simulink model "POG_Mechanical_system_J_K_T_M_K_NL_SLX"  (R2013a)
settings: Solver=ode45  StartTime=0.0  StopTime=10.0  MaxStep=0.001  RelTol=1e-3
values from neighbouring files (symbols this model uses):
  b_1 = 1*Nm/(10*rpm)    (= 0.954929658551)    [POG_Mechanical_system_J_K_T_M_K_Par_SLX_m.m]    (also in POG_Mechanical_system_J_K_T_M_K_SLX_m.m = 1; POG_Mechanical_system_J_K_T_M_K_SuperBlock_SLX_m.m = 1; POG_Mechanical_system_J_K_T_M_K_NL_SLX_m.m)
  F_out = [-K_1*x_b -x_b x_b K_1*x_b]    [POG_Mechanical_system_J_K_T_M_K_NL_SLX_m.m]
  J = 1*kg*(30*cm)^2    (= 0.09)    [POG_Mechanical_system_J_K_T_M_K_Par_SLX_m.m]    (also in POG_Mechanical_system_J_K_T_M_K_SLX_m.m = 1; POG_Mechanical_system_J_K_T_M_K_SuperBlock_SLX_m.m = 1; POG_Mechanical_system_J_K_T_M_K_NL_SLX_m.m)
  K_2 = 20*Newton/(1*cm)    (= 2000)    [POG_Mechanical_system_J_K_T_M_K_Par_SLX_m.m]    (also in POG_Mechanical_system_J_K_T_M_K_SLX_m.m = 1; POG_Mechanical_system_J_K_T_M_K_SuperBlock_SLX_m.m = 1; POG_Mechanical_system_J_K_T_M_K_NL_SLX_m.m)
  Nc = 30*Newton    (= 30)    [POG_Mass_Linear_Control_SLX_m.m]    (also in POG_Mechanical_system_J_K_T_M_K_NL_SLX_m.m = 2)
  P_2_0 = 0    [POG_Mechanical_system_J_K_T_M_K_Par_SLX_m.m]    (also in POG_Mechanical_system_J_K_T_M_K_SLX_m.m; POG_Mechanical_system_J_K_T_M_K_SuperBlock_SLX_m.m; POG_Mechanical_system_J_K_T_M_K_NL_SLX_m.m)
  Ph_T = pi/2    (= 1.57079632679)    [POG_Mechanical_system_J_K_T_M_K_NL_SLX_m.m]
  R = 40*cm    (= 0.4)    [POG_Mechanical_system_J_K_T_M_K_Par_SLX_m.m]    (also in POG_Mechanical_system_J_K_T_M_K_SLX_m.m = 1; POG_Mechanical_system_J_K_T_M_K_SuperBlock_SLX_m.m = 1; POG_Mechanical_system_J_K_T_M_K_NL_SLX_m.m)
  T = 10*Nm    (= 10)    [POG_Mechanical_system_J_K_T_M_K_Par_SLX_m.m]    (also in POG_Mechanical_system_J_K_T_M_K_SLX_m.m; POG_Mechanical_system_J_K_T_M_K_SuperBlock_SLX_m.m; POG_Mechanical_system_J_K_T_M_K_NL_SLX_m.m = 2)
  Ts = Tfin/Nr_Ts_Points    (= 0.0025)    [POG_Mechanical_system_J_K_T_M_K_Par_SLX_m.m]    (also in POG_Mechanical_system_J_K_T_M_K_SLX_m.m = 0.005; POG_Mechanical_system_J_K_T_M_K_SuperBlock_SLX_m.m = 0.005; POG_Mass_Linear_Control_SLX_m.m; POG_Mechanical_system_J_K_T_M_K_NL_SLX_m.m)
  v_d = 0    [POG_Mechanical_system_J_K_T_M_K_Par_SLX_m.m]    (also in POG_Mechanical_system_J_K_T_M_K_SLX_m.m; POG_Mechanical_system_J_K_T_M_K_SuperBlock_SLX_m.m; POG_Mechanical_system_J_K_T_M_K_NL_SLX_m.m)
  Vx0 = 0    [POG_Mechanical_system_J_K_T_M_K_NL_SLX_m.m]
  w_T = 2*pi*1    (= 6.28318530718)    [POG_Mechanical_system_J_K_T_M_K_NL_SLX_m.m]
  x_6_0 = 0    [POG_Mechanical_system_J_K_T_M_K_Par_SLX_m.m]    (also in POG_Mechanical_system_J_K_T_M_K_SLX_m.m; POG_Mechanical_system_J_K_T_M_K_SuperBlock_SLX_m.m; POG_Mechanical_system_J_K_T_M_K_NL_SLX_m.m)
  x_9_0 = 0    [POG_Mechanical_system_J_K_T_M_K_Par_SLX_m.m]    (also in POG_Mechanical_system_J_K_T_M_K_SLX_m.m; POG_Mechanical_system_J_K_T_M_K_SuperBlock_SLX_m.m; POG_Mechanical_system_J_K_T_M_K_NL_SLX_m.m)
  X_in = [  -2*x_b -x_b x_b   2*x_b]    [POG_Mechanical_system_J_K_T_M_K_NL_SLX_m.m]
undefined symbols (not defined in the file or in its folder): b, m

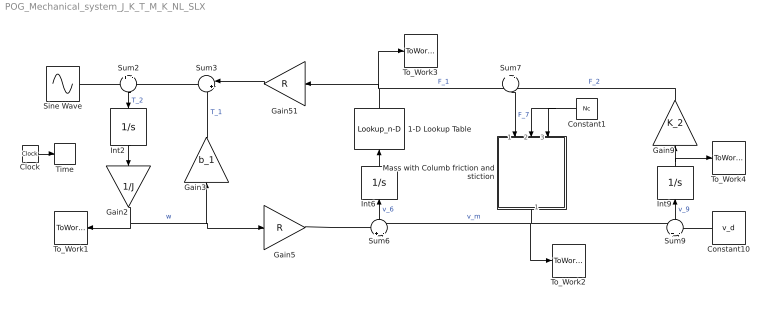
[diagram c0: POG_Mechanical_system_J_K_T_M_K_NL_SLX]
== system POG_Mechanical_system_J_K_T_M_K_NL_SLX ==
  1-D Lookup Table : Lookup_n-D  NumberOfTableDimensions=1  BreakpointsForDimension1=X_in  Table=F_out  RndMeth=Simplest
  Clock : Clock
  Constant1 : Constant  Value=Nc
  Constant10 : Constant  Value=v_d
  Gain2 : Gain  Gain=1/J
  Gain3 : Gain  Gain=b_1
  Gain5 : Gain  Gain=R
  Gain51 : Gain  Gain=R
  Gain9 : Gain  Gain=K_2
  Int2 : Integrator  InitialCondition=P_2_0
  Int6 : Integrator  InitialCondition=x_6_0
  Int9 : Integrator  InitialCondition=x_9_0
  Mass with Columb friction and stiction : Subsystem
  Sine Wave : Sin  Amplitude=T  Frequency=w_T  Phase=Ph_T  SampleTime=0
  Sum{2,6..7,9} (4 alike) : Sum  Inputs=+|-
  Sum3 : Sum  Inputs=|++
  Time : ToWorkspace  VariableName=t  SampleTime=Ts
  To_Work1 : ToWorkspace  VariableName=w_1  SampleTime=Ts
  To_Work2 : ToWorkspace  VariableName=w_m  SampleTime=Ts
  To_Work3 : ToWorkspace  VariableName=F_1  SampleTime=Ts
  To_Work4 : ToWorkspace  VariableName=x  SampleTime=Ts
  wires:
  Sine Wave/1 -> Sum2/1
  Sum3/1 -> Sum2/2
  Gain2/1 -> To_Work1/1, Gain3/1, Gain5/1  "w"
  Sum2/1 -> Int2/1  "T_2"
  Int2/1 -> Gain2/1
  Gain51/1 -> Sum3/1
  Gain3/1 -> Sum3/2  "T_1"
  Gain5/1 -> Sum6/1
  1-D Lookup Table/1 -> To_Work3/1, Gain51/1, Sum7/1  "F_1"
  Mass with Columb friction and stiction/1(Vx) -> Sum6/2, To_Work2/1, Sum9/1  "v_m"
  Sum6/1 -> Int6/1  "v_6"
  Int6/1 -> 1-D Lookup Table/1
  Sum7/1 -> Mass with Columb friction and stiction/1(F)  "F_7"
  Gain9/1 -> Sum7/2  "F_2"
  Constant10/1 -> Sum9/2
  Sum9/1 -> Int9/1  "v_9"
  Int9/1 -> To_Work4/1, Gain9/1
  Clock/1 -> Time/1
  Constant1/1 -> Mass with Columb friction and stiction/3(Ns), Mass with Columb friction and stiction/2(Nc)

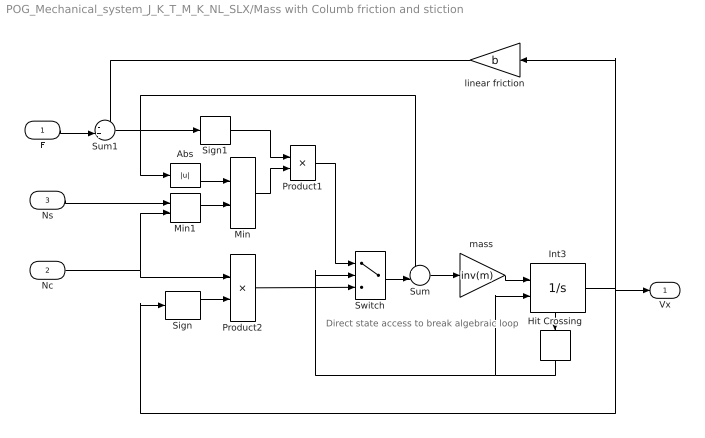
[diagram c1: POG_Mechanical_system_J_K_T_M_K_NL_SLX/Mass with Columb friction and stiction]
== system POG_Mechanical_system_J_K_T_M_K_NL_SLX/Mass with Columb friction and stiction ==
  note: Direct state access to break algebraic loop
  F : Inport
  Nc : Inport  Port=2
  Ns : Inport  Port=3
  Abs : Abs
  Hit Crossing : HitCross
  Int3 : Integrator  ExternalReset=rising  InitialCondition=Vx0  ShowStatePort=on
  Min : MinMax  Inputs=2
  Min1 : MinMax  Function=max  Inputs=2
  Product1 : Product
  Product2 : Product
  Sign : Signum
  Sign1 : Signum
  Sum : Sum  Inputs=+-|
  Sum1 : Sum  Inputs=-+|
  Switch : Switch  Threshold=0.5
  linear friction : Gain  Gain=b
  "mass " : Gain  Gain=inv(m)
  Vx : Outport  InitialOutput=0
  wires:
  F/1 -> Sum1/2
  linear friction/1 -> Sum1/1
  Ns/1 -> Min1/1
  Min1/1 -> Min/2
  Abs/1 -> Min/1
  Min/1 -> Product1/2
  Sign1/1 -> Product1/1
  Sign/1 -> Product2/2
  Nc/1 -> Min1/2, Product2/1
  Product2/1 -> Switch/3
  Int3/1 -> linear friction/1, Sign/1, Vx/1
  Int3/State -> Hit Crossing/1
  "mass "/1 -> Int3/1
  Sum/1 -> "mass "/1
  Sum1/1 -> Sign1/1, Abs/1, Sum/1
  Hit Crossing/1 -> Int3/2, Switch/2
  Switch/1 -> Sum/2
  Product1/1 -> Switch/1
